(* Logix 5000 Routine export Limit; software revision 20.01 *)

TYPE Limit :
STRUCT
   test : REAL;
   high : REAL;
   low : REAL;
   default : REAL;
END_STRUCT
END_TYPE

VAR_GLOBAL   (* controller tags *)
   Limit : Limit := (test := 1.68155816e-044, high := 1.39989717e-042); {access Read Only}
END_VAR

PROGRAM DET_COM

ROUTINE Limit   (* ladder *)
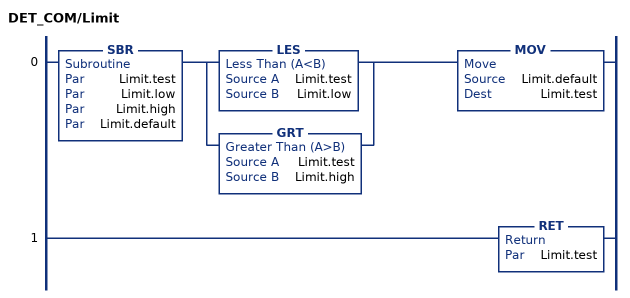
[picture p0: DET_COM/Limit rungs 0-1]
   0: SBR(Limit.test,Limit.low,Limit.high,Limit.default)[LES(Limit.test,Limit.low) ,GRT(Limit.test,Limit.high) ]MOV(Limit.default,Limit.test);
   1: RET(Limit.test);
END_ROUTINE
END_PROGRAM
